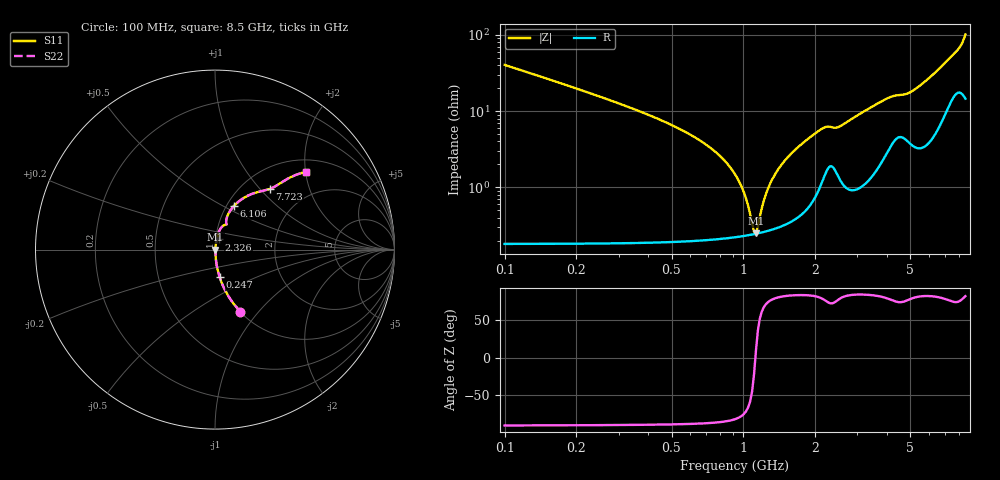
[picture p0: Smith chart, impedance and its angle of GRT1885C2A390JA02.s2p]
!Murata Part Number: GRT1885C2A390JA02
!These Parameters are Measured in Series Mode Connection
!Data Generated on Jun 19, 2026
!  o--ll--o
!Port1  Port2
!  o------o
!Operation Temp=25[degC], DC Bias Voltage=0[V]
!Freq. Start=100[MHz] Stop=9[GHz] 401[Steps]
# Hz S RI R 50
!Freq.(Hz) S11(Real) S11(Imag) S21(Real) S21(Imag) S12(Real) S12(Imag) S22(Real) S22(Imag)
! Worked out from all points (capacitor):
!   401 points, 100 MHz to 8.5 GHz, reference 50 ohm
!   read as one part in series: C = 39 pF near 142 MHz
!   lowest |Z| = 250 mohm at 1.129 GHz (marker M1)
!   series resonance near 1.122 GHz, so ESL is about 520 pH
!   S11 on the Smith chart (normalised r, x): 100 MHz: 1.00, -0.81; 247 MHz: 1.00, -0.31; 2.326 GHz: 1.04, +0.12; 6.106 GHz: 1.08, +0.57; 7.723 GHz: 1.33, +1.14; 8.5 GHz: 1.29, +2.01
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1e8  0.142 -0.3468  0.858 0.3468  0.858 0.3468  0.142 -0.3468
2.47e8  0.0259 -0.1531  0.9741 0.1531  0.9741 0.1531  0.0259 -0.1531
8.56e8  0.00255 -0.0202  0.9975 0.0202  0.9975 0.0202  0.00255 -0.0202
9.61e8  0.00237 -0.0115  0.9976 0.0115  0.9976 0.0115  0.00237 -0.0115
1.024e9  0.00236 -0.0068  0.9976 0.0068  0.9976 0.0068  0.00236 -0.0068
1.087e9  0.0024 -0.00237  0.9976 0.00237  0.9976 0.00237  0.0024 -0.00237
1.129e9  0.00245 0.000453  0.9976 -0.000453  0.9976 -0.000453  0.00245 0.000453
1.297e9  0.00285 0.011  0.9972 -0.011  0.9972 -0.011  0.00285 0.011
1.507e9  0.00377 0.023  0.9962 -0.023  0.9962 -0.023  0.00377 0.023
1.969e9  0.00912 0.0481  0.9909 -0.0481  0.9909 -0.0481  0.00912 0.0481
2.326e9  0.0219 0.0565  0.9781 -0.0565  0.9781 -0.0565  0.0219 0.0565
2.494e9  0.0171 0.0582  0.9829 -0.0582  0.9829 -0.0582  0.0171 0.0582
2.914e9  0.0157 0.0806  0.9843 -0.0806  0.9843 -0.0806  0.0157 0.0806
3.712e9  0.0341 0.1217  0.9659 -0.1217  0.9659 -0.1217  0.0341 0.1217
4.3e9  0.0601 0.139  0.9399 -0.139  0.9399 -0.139  0.0601 0.139
4.888e9  0.0623 0.1505  0.9377 -0.1505  0.9377 -0.1505  0.0623 0.1505
5.707e9  0.081 0.2106  0.919 -0.2106  0.919 -0.2106  0.081 0.2106
6.106e9  0.1061 0.2436  0.8939 -0.2436  0.8939 -0.2436  0.1061 0.2436
7.114e9  0.2195 0.315  0.7805 -0.315  0.7805 -0.315  0.2195 0.315
7.723e9  0.3061 0.3383  0.6939 -0.3383  0.6939 -0.3383  0.3061 0.3383
8.164e9  0.3816 0.3815  0.6184 -0.3815  0.6184 -0.3815  0.3816 0.3815
8.5e9  0.5064 0.4326  0.4936 -0.4326  0.4936 -0.4326  0.5064 0.4326
